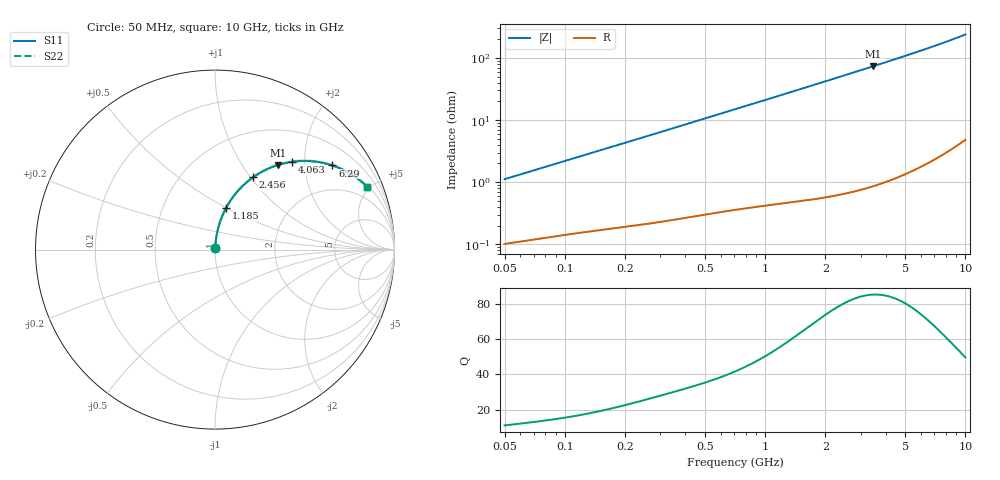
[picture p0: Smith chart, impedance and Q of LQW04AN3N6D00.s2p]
!Murata Part Number: LQW04AN3N6D00
!These Parameters are Measured in Series Mode Connection
!  o--[Z]--o
!Port1  Port2
!  o-------o
!Freq. Start=50[MHz] Stop=10[GHz], 401[Steps]
# Hz S RI R 50
!Freq.(Hz)	S 11(Real)	S 11(Imag)	S 21(Real)	S 21(Imag)	S 12(Real)	S 12(Imag)	S 22(Real)	S 22(Imag)
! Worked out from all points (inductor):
!   401 points, 50 MHz to 10 GHz, reference 50 ohm
!   read as one part in series: L = 3.52 nH near 51.34 MHz
!   highest Q = 85.3 at 3.466 GHz (marker M1), where L = 3.37 nH
!   S11 on the Smith chart (normalised r, x): 50 MHz: 1.00, +0.02; 1.185 GHz: 1.01, +0.50; 2.456 GHz: 1.01, +1.03; 4.063 GHz: 1.02, +1.73; 6.29 GHz: 1.04, +2.76; 10 GHz: 1.10, +4.77
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5e7  0.00114 0.0111  0.9989 -0.0111  0.9989 -0.0111  0.00114 0.0111
1.214486e8  0.00223 0.0263  0.9978 -0.0263  0.9978 -0.0263  0.00223 0.0263
1.956524e8  0.00363 0.0418  0.9964 -0.0418  0.9964 -0.0418  0.00363 0.0418
2.949953e8  0.00618 0.0624  0.9938 -0.0624  0.9938 -0.0624  0.00618 0.0624
4.689809e8  0.0126 0.0978  0.9874 -0.0978  0.9874 -0.0978  0.0126 0.0978
7.071068e8  0.025 0.1447  0.975 -0.1447  0.975 -0.1447  0.025 0.1447
9.215873e8  0.0397 0.1852  0.9603 -0.1852  0.9603 -0.1852  0.0397 0.1852
1.185319e9  0.0619 0.2322  0.9381 -0.2322  0.9381 -0.2322  0.0619 0.2322
1.445853e9  0.0879 0.2752  0.9121 -0.2752  0.9121 -0.2752  0.0879 0.2752
1.717543e9  0.1184 0.3159  0.8816 -0.3159  0.8816 -0.3159  0.1184 0.3159
2.067491e9  0.1618 0.3617  0.8382 -0.3617  0.8382 -0.3617  0.1618 0.3617
2.455993e9  0.2135 0.4036  0.7865 -0.4036  0.7865 -0.4036  0.2135 0.4036
2.917498e9  0.2769 0.4416  0.7231 -0.4416  0.7231 -0.4416  0.2769 0.4416
3.465724e9  0.3517 0.4717  0.6483 -0.4717  0.6483 -0.4717  0.3517 0.4717
4.062795e9  0.4289 0.489  0.5711 -0.489  0.5711 -0.489  0.4289 0.489
4.171863e9  0.4423 0.4908  0.5577 -0.4908  0.5577 -0.4908  0.4423 0.4908
5.088839e9  0.5454 0.4917  0.4546 -0.4917  0.4546 -0.4917  0.5454 0.4917
6.290134e9  0.6537 0.4689  0.3463 -0.4689  0.3463 -0.4689  0.6537 0.4689
7.086521e9  0.7103 0.4462  0.2897 -0.4462  0.2897 -0.4462  0.7103 0.4462
8.090191e9  0.7678 0.414  0.2322 -0.414  0.2322 -0.414  0.7678 0.414
9.236013e9  0.8185 0.3762  0.1815 -0.3762  0.1815 -0.3762  0.8185 0.3762
1e10  0.8454 0.3515  0.1546 -0.3515  0.1546 -0.3515  0.8454 0.3515
